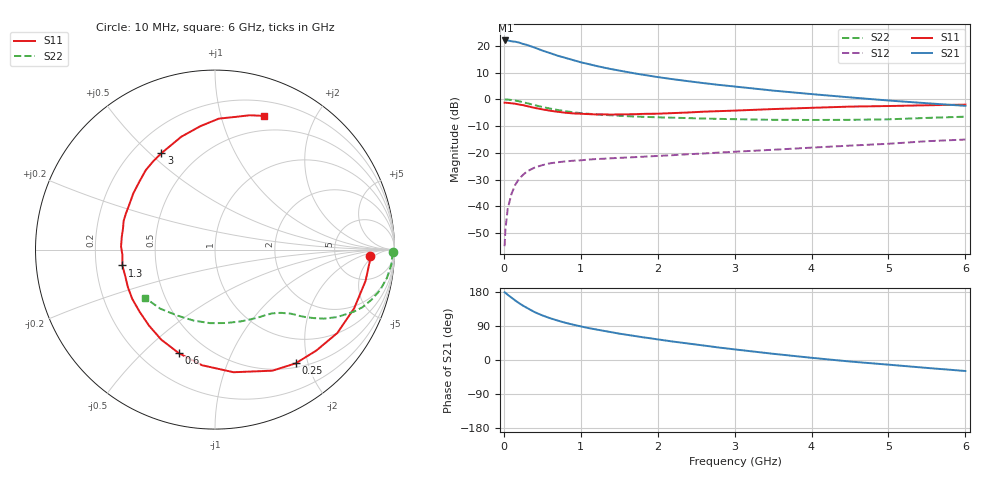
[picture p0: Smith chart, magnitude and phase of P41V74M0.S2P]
! SIEMENS Small Signal Semiconductors
! BFP182
! Si NPN RF Bipolar Junction Transistor in SOT143
! VCE = 1.75 V  IC = 4 mA
! Common Emitter S-Parameters:  March  1996
# GHz  S  MA  R  50
!  f  S11  S21  S12  S22
! GHz  MAG  ANG  MAG  ANG  MAG  ANG  MAG  ANG
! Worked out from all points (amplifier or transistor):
!   36 points, 10 MHz to 6 GHz, reference 50 ohm
!   highest |S21| = 22.0 dB at 20 MHz (marker M1)
!   |S21| within 3 dB of that: start of sweep to 430.4 MHz
!   unconditionally stable (mu >= 1): 1.677 GHz to 5.66 GHz
!   at 250 MHz: K = 0.19, MSG = 24.5 dB, |S12| = -28.2 dB
!   at 1.4 GHz: K = 0.89, MSG = 16.7 dB, |S12| = -22.0 dB
!   at 6 GHz: K = 0.95, MSG = 6.3 dB, |S12| = -15.0 dB
!   S11 on the Smith chart (normalised r, x): 10 MHz: 13, -4; 250 MHz: 0.56, -1.80; 600 MHz: 0.35, -0.65; 1.3 GHz: 0.31, -0.08; 3 GHz: 0.32, +0.54; 6 GHz: 0.34, +1.38
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0.01  0.8637 -2.5  12.4 178.7  0.0018 84.5  0.9916 -0.9
0.02  0.8643 -4.6  12.57 177.4  0.0036 90.1  0.9883 -1.9
0.05  0.8567 -11.8  12.57 172.1  0.0089 85.9  0.9862 -4.8
0.15  0.8249 -34.3  11.89 156.8  0.0255 70.5  0.9471 -13.8
0.2  0.7969 -44.9  11.45 149.7  0.0328 66.3  0.9161 -17.7
0.25  0.7767 -54.7  10.81 143.3  0.0388 61.5  0.8829 -21.3
0.3  0.7468 -64.6  10.37 137.6  0.0448 57.1  0.847 -24.1
0.4  0.691 -81.4  9.252 126.4  0.0529 50.2  0.7777 -28.9
0.5  0.6483 -96.4  8.142 117.7  0.0588 44.1  0.7179 -32.4
0.6  0.6113 -109.2  7.31 110.4  0.0636 40.5  0.6707 -34.7
0.7  0.5844 -120.8  6.52 104.0  0.0666 37.3  0.6313 -36.6
0.8  0.5608 -131.0  5.945 98.2  0.069 35.0  0.5989 -38.1
0.9  0.5445 -140.4  5.41 93.3  0.0711 33.2  0.5724 -39.2
1.1  0.5286 -156.7  4.555 84.3  0.0747 30.5  0.5361 -41.5
1.3  0.5236 -170.3  3.913 76.9  0.0775 28.9  0.5112 -43.6
1.7  0.5257 167.2  3.05 63.4  0.0829 28.1  0.476 -48.3
2.2  0.5524 145.5  2.37 48.6  0.0904 27.8  0.4527 -55.6
3  0.6144 119.1  1.733 28.0  0.1047 26.7  0.4248 -70.4
3.5  0.6564 106.6  1.454 16.4  0.114 25.6  0.4137 -81.4
4.5  0.7301 88.3  1.085 -4.0  0.1362 22.0  0.4131 -106.6
5.5  0.7731 75.5  0.844 -20.9  0.1646 17.6  0.4487 -132.8
6  0.7942 69.7  0.754 -29.0  0.177 13.5  0.4733 -145.4
